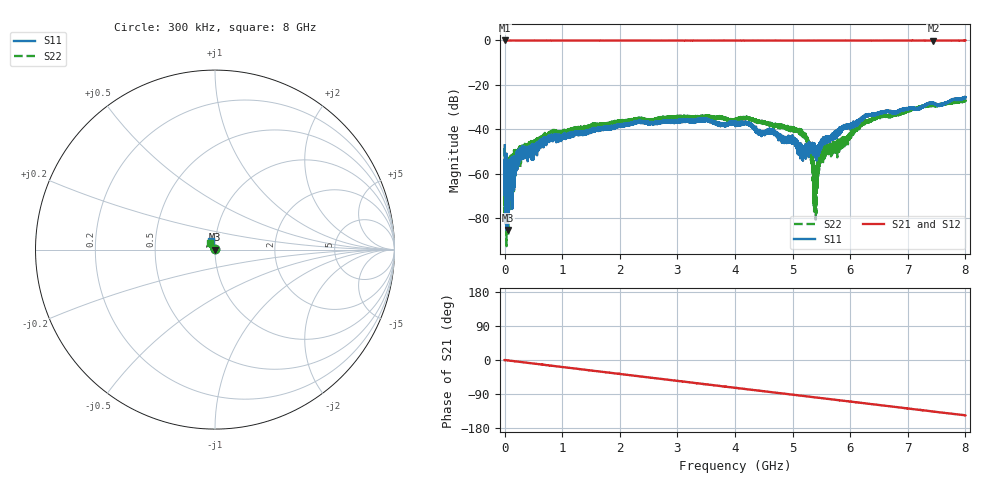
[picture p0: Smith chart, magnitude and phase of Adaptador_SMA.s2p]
#  HZ  S  DB  R  50.00
! Rohde & Schwarz ZVA/B
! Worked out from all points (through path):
!   30000 points, 300 kHz to 8 GHz, reference 50 ohm
!   highest |S21| = 0.02 dB at 2.167 MHz (marker M1); lowest = 0.0 dB at 7.445 GHz (marker M2)
!   group delay of S21, straight-line fit = 50.7 ps
!   lowest |S11| = -85.1 dB at 57.9 MHz (marker M3), VSWR 1.00, Z = 50 + j0.000646 ohm
!   |S11| at or under -10 dB: start of sweep to end of sweep
!   |S22| runs from -92.5 to -26.7 dB; largest |S21 - S12| = 0.0045
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300000  -47.09 117.2  -0.01 -0.1  -0.01 -0.1  -48.28 56.6
2166659  -56.12 142.1  0.02 0.0  0.01 0.0  -60.77 -45.4
4.029983e7  -63.21 93.1  -0.00 -0.7  -0.01 -0.8  -60.82 -156.3
5.789976e7  -85.12 6.7  -0.01 -1.1  -0.00 -1.0  -55.15 91.9
1.666993e8  -54.11 76.5  -0.01 -3.1  -0.01 -3.1  -52.16 63.8
2.954988e8  -50.77 65.3  -0.01 -5.4  -0.02 -5.4  -47.63 79.0
8.368298e8  -44.09 65.7  -0.02 -15.5  -0.02 -15.4  -41.94 54.0
1.333628e9  -41.37 69.9  -0.02 -24.6  -0.02 -24.5  -39.16 50.3
2.666956e9  -36.75 41.9  -0.02 -49.0  -0.03 -48.9  -34.92 34.0
4.000283e9  -37.40 1.9  -0.03 -73.3  -0.03 -73.2  -35.91 26.3
4.647747e9  -41.34 -16.0  -0.03 -85.1  -0.02 -85.1  -38.02 12.6
5.125879e9  -48.49 -34.2  -0.02 -93.8  -0.03 -93.8  -41.42 4.4
5.251211e9  -49.06 -102.0  -0.03 -96.1  -0.03 -96.1  -44.02 15.2
5.333611e9  -46.95 -118.8  -0.02 -97.6  -0.03 -97.5  -55.34 21.6
5.366411e9  -50.47 -129.1  -0.02 -98.2  -0.02 -98.1  -61.42 51.1
5.397878e9  -50.34 -165.3  -0.02 -98.7  -0.02 -98.7  -60.42 -26.9
5.478144e9  -46.73 171.8  -0.02 -100.1  -0.03 -100.2  -53.97 -114.6
5.56081e9  -44.95 152.3  -0.03 -101.7  -0.03 -101.7  -49.67 -103.4
6.202674e9  -35.08 151.3  -0.03 -113.3  -0.03 -113.3  -37.49 174.7
6.666939e9  -32.17 144.6  -0.02 -121.8  -0.03 -121.8  -34.06 161.4
7.444536e9  -28.30 128.1  -0.04 -136.0  -0.03 -136.0  -29.12 137.5
8e9  -25.44 117.8  -0.02 -146.0  -0.03 -146.0  -26.86 127.0
